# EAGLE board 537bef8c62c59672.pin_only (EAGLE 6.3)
REV: A

Size 53.34 x 40.64 mm. Coordinates in mm from the lower left corner, seen from the top.
Outline: 2.54,40.64 50.8,40.64 arc-90 53.34,38.1 53.34,2.54 arc-90 50.8,0 2.54,0 arc-90 0,2.54 0,38.1 arc-90 2.54,40.64
Copper layers (1*16): Top 0.035mm / dielectric 1.5mm / Bottom 0.035mm
Design rules "adafruit *": minimum track width 10mil, minimum drill 15.5mil, track to track 8mil, track to pad 8mil, pad to pad 8mil, via to via 8mil, smd to smd 8mil, copper to edge 10mil, drill to drill 8mil, minimum pad ring 10mil, minimum via ring 8mil, stop-mask expansion 4mil, vias tented up to drill 20mil, thermal gap 10mil
tRestrict: area 29.1,23.7 to 29.2,24.6; area 28.1,24 to 28.2,24.9; area 30.4,22.7 to 31.2,22.9; area 30.4,21.7 to 31.2,21.8; area 30.5,19.3 to 31.4,19.4; area 30.5,18.8 to 31.4,18.9

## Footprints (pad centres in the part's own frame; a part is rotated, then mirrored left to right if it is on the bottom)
CELEC_3.5MM_8MM = drill 0.813 pad 1.6: + -1.778,0 | drill 0.813 pad 1.6 octagon: - 1.778,0
0805-NO = smd 1.3 x 1.5: 1 -0.95,0; 2 0.95,0
DCJACK_2MM_SMT = smd 2.4 x 2: GND 0,-5.5; GNDBREAK 6.2,-5.5; PWR 0,5.5; PWR2 6.2,5.5 | hole 1.6: 0,0 | hole 1.8: 4.5,0
SOD-323 = smd 1.35 x 0.8: A 1.27,0; C -1.27,0
_0805 = smd 1.2 x 1.3: 1 -1.016,0; 2 1.016,0
FIDUCIAL_1MM = smd 1 x 1: 1 0,0
TERMBLOCK_1X2-3.5MM = drill 1 pad 2.184: 1 1.8,0; 2 -1.7,0
1X14_ROUND70 = drill 1 pad 1.676 square: 1 -16.51,0 | drill 1 pad 1.676: 2 -13.97,0; 3 -11.43,0; 4 -8.89,0; 5 -6.35,0; 6 -3.81,0; 7 -1.27,0; 8 1.27,0; 9 3.81,0; 10 6.35,0; 11 8.89,0; 12 11.43,0; 13 13.97,0; 14 16.51,0
TO252 = smd 1 x 1.6: 1 -2.28,-4.8; 2 2.28,-4.8 | smd 5.4 x 6.2: 3 0,2.5
SOT23-WIDE = smd 1 x 1.2: 1 -0.95,-1; 2 0.95,-1; 3 0,1
_0805MP = smd 1.2 x 1.3: 1 -1.016,0; 2 1.016,0
SOLDERJUMPER_ARROW_NOPASTE = smd 0.762 x 1.524: 1 -1.016,0; 2 1.016,0
TQFN44_7MM = smd 0.25 x 1.05: 1 -2.5,-3.475; 2 -2,-3.475; 3 -1.5,-3.475; 4 -1,-3.475; 5 -0.5,-3.475; 6 0,-3.475; 7 0.5,-3.475; 8 1,-3.475; 9 1.5,-3.475; 10 2,-3.475; 11 2.5,-3.475; 23 2.5,3.475; 24 2,3.475; 25 1.5,3.475; 26 1,3.475; 27 0.5,3.475; 28 0,3.475; 29 -0.5,3.475; 30 -1,3.475; 31 -1.5,3.475; 32 -2,3.475; 33 -2.5,3.475 | smd 1.05 x 0.25: 12 3.475,-2.5; 13 3.475,-2; 14 3.475,-1.5; 15 3.475,-1; 16 3.475,-0.5; 17 3.475,0; 18 3.475,0.5; 19 3.475,1; 20 3.475,1.5; 21 3.475,2; 22 3.475,2.5; 34 -3.475,2.5; 35 -3.475,2; 36 -3.475,1.5; 37 -3.475,1; 38 -3.475,0.5; 39 -3.475,0; 40 -3.475,-0.5; 41 -3.475,-1; 42 -3.475,-1.5; 43 -3.475,-2; 44 -3.475,-2.5 | smd 4.7 x 4.7: THERMAL 0,0
SOT23-5 = smd 0.55 x 1.2: 1 -0.95,-1.3; 2 0,-1.3; 3 0.95,-1.3; 4 0.95,1.3; 5 -0.95,1.3
MOUNTINGHOLE_2.5_PLATED_THICK = drill 2.5 pad 4: P$1 0,0
TRIMPOT_100MILPTH = drill 0.813 long: A 2.54,1.27; E -2.54,1.27; S 0,1.27
TERMBLOCK_1X3-3.5MM = drill 1 pad 2.184: 1 3.55,0; 2 0.05,0; 3 -3.45,0
4UCONN_19269 = smd 2 x 2.5: 1 2.5,-3.5; 2 11.7,-3.5; 3 4.3,3.5 | smd 2.5 x 2: 4 15.8,0.75 | smd 1.2 x 2.5: 5 1.5,3.5 | hole 2: 3.5,0; 10.5,0

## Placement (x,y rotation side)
C1  330µF  [CELEC_3.5MM_8MM]  41.68,36.38 270 top
C2  10µF  [0805-NO]  12.45,26.59 90 top
C3  10µF  [0805-NO]  46.93,34.44 270 top
C4  10µF  [0805-NO]  19.32,26.59 270 top
C5  2.2µF  [0805-NO]  21.53,15.09 270 top
C6  0.1µF  [0805-NO]  38.92,18.92 0 top
C7  470pF  [0805-NO]  44.13,14.22 270 top
C8  0.1µF  [0805-NO]  38.92,15.11 0 top
C9  470pF  [0805-NO]  44.13,18.16 90 top
C10  0.1µF  [0805-NO]  29.43,27.18 180 top
C11  0.1µF  [0805-NO]  28.92,13.51 0 top
C13  0.1µF  [0805-NO]  38.92,22.23 0 top
C15  0.1µF  [0805-NO]  38.92,26.42 0 top
C16  470pF  [0805-NO]  44.13,27.18 90 top
C17  470pF  [0805-NO]  44.13,23.24 270 top
C22  0.47µF  [0805-NO]  15.8,23 0 top
C23  0.47µF  [0805-NO]  15.8,20.97 0 top
CN1  2.1mm  [DCJACK_2MM_SMT]  15.59,38.72 270 top
D1  1N4148  [SOD-323]  23.97,6.6 90 top
D2  1N4148  [SOD-323]  36.29,7.24 90 top
D3  1N4148  [SOD-323]  34.51,7.24 90 top
D4  1N4148  [SOD-323]  32.61,7.24 90 top
FB1  MPZ2012S221A  [_0805]  10.12,25.32 90 top
FB2  MPZ2012S221A  [_0805]  42.1,18.16 90 top
FB3  MPZ2012S221A  [_0805]  42.1,14.22 90 top
FB4  MPZ2012S221A  [_0805]  42.1,23.24 270 top
FB5  MPZ2012S221A  [_0805]  42.1,27.18 270 top
FID1  FIDUCIAL""  [FIDUCIAL_1MM]  51.97,34.22 0 top
FID2  FIDUCIAL""  [FIDUCIAL_1MM]  6.6,2.29 0 top
J1  3.5mm  [TERMBLOCK_1X2-3.5MM]  26.38,36.56 180 top
J2  SPKRIGHT  [TERMBLOCK_1X2-3.5MM]  49.59,15.75 90 top
J3  SPKLEFT  [TERMBLOCK_1X2-3.5MM]  49.59,25.4 90 top
JP2  [1X14_ROUND70]  26.67,2.54 0 top
Q1  AOD417  [TO252]  33.88,34.71 0 top
Q2  BSS138  [SOT23-WIDE]  14.19,10.29 90 top
Q3  BS138  [SOT23-WIDE]  14.19,6.73 90 top
Q4  BSS138  [SOT23-WIDE]  26.77,8.64 0 top
R1  10K  [0805-NO]  17.05,14.06 0 top
R2  10K  [_0805MP]  26.77,11.71 0 top
R3  10K  [0805-NO]  16.86,6.73 270 top
R4  10K  [0805-NO]  19.02,6.63 90 top
R5  10K  [0805-NO]  21.18,6.63 90 top
R6  20K  [0805-NO]  20.76,22.78 270 top
R7  20K  [0805-NO]  20.76,18.99 90 top
R8  20K  [0805-NO]  18.8,22.81 270 top
R9  20K  [0805-NO]  18.77,18.96 270 top
R10  10K  [_0805MP]  24.23,27.05 90 top
R11  10K  [_0805MP]  22.19,27.05 90 top
R12  10K  [0805-NO]  22.8,9.53 180 top
R14  10K  [_0805MP]  29.81,10.7 90 top
R15  10K  [_0805MP]  28.92,5.87 180 top
SJ1  [SOLDERJUMPER_ARROW_NOPASTE]  6.33,29.36 180 bottom
SJ3  [SOLDERJUMPER_ARROW_NOPASTE]  42.39,7.24 270 top
SJ4  [SOLDERJUMPER_ARROW_NOPASTE]  39.59,7.24 270 top
SJ5  [SOLDERJUMPER_ARROW_NOPASTE]  19.27,9.53 0 top
U1  MAX9744  [TQFN44_7MM]  27.4,20.57 180 top
U2  MIC5225-3.3  [SOT23-5]  15.86,26.59 270 top
U$28  [ADAFRUIT_TEXT_20MM]  39.5,3.56 0 bottom
U$29  MOUNTINGHOLE2.5_THICK  [MOUNTINGHOLE_2.5_PLATED_THICK]  2.54,2.54 0 top
U$32  [ADAFRUIT_5MM]  44.58,3.68 0 top
U$38  MOUNTINGHOLE2.5_THICK  [MOUNTINGHOLE_2.5_PLATED_THICK]  50.8,2.54 0 top
U$39  MOUNTINGHOLE2.5_THICK  [MOUNTINGHOLE_2.5_PLATED_THICK]  2.54,38.1 0 top
U$40  MOUNTINGHOLE2.5_THICK  [MOUNTINGHOLE_2.5_PLATED_THICK]  50.8,38.1 0 top
U$41  [ICON_POSITIVE_CENTER-M]  7.46,37.48 270 top
U$42  [ICON_PLUS]  29.17,32.09 0 top
U$43  [ICON_MINUS]  23.24,32.09 0 top
U$47  [ICON_MINUS]  8.21,27.79 90 top
U$50  [ICON_PLUS]  52.16,30.5 0 top
U$51  [ICON_MINUS]  52.13,20.7 90 top
U$52  [ICON_PLUS]  52.13,10.78 0 top
VR1  Must be <1Kohm  [TRIMPOT_100MILPTH]  4.96,8.82 180 top
X1  3.5mm  [TERMBLOCK_1X3-3.5MM]  3.63,27.69 270 top
X2  3.5mm  [4UCONN_19269]  0,16.89 0 top

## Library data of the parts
C1-C9 C13 C15-C17 C22 C23 CN1 D1-D4 FB1-FB5 J1-J3 Q1-Q4 R1-R12 U1 U2 U$28 U$32 U$41-U$43 U$47 U$50-U$52 VR1 X1 X2 = microbuilder
C10 C11 JP2 R14 R15 = microbuilder; AUTHOR: K. Townsend
FID1 FID2 SJ3-SJ5 U$29 U$38-U$40 = microbuilder; BOM: EXCLUDE
SJ1 = microbuilder; AUTHOR: K. Townsend; BOM: EXCLUDE

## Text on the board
tPlace: 12V | R | Left | L | MAX9744 / Class D | 4-8ΩBTL | Analog | Right | Pot. Vol | AD1 | AD2 | RIN | AGND | SCL | SHDN | SYNCO | AD1 | GND | LIN | SDA | Vi2c | MUTE | SYNC | AD2 | VDD
bPlace: MAX9744 20W Class D | Stereo Amplifier | 5-14VDC / Max! | For I2C Mode (default) / Keep Analog, AD1 & AD2 jumper open / Connect Vi2c to 3-5V. Addr is 0x4B / Close either AD1 or AD2 to change addr / Write 0x0-0x3F to I2C to set volume | For Analog mode / Close Analog, AD1 & AD2 jumpers / Or connect SCL/AD1/AD2 pins to Gnd / Connect 1K pot to three pads | BTL Outputs | Power per Channel | 13W @ 14V->8Ω / 22W @ 14V->4Ω | 10W @ 12V->8Ω / 17W @ 12V->4Ω | 1.8W @ 5V->8Ω / 3.6W @ 5V->4Ω

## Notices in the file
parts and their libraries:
microbuilder: This work is placed in the public domain, and may be freely used for commercial and non-commercial work with the following conditions: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
